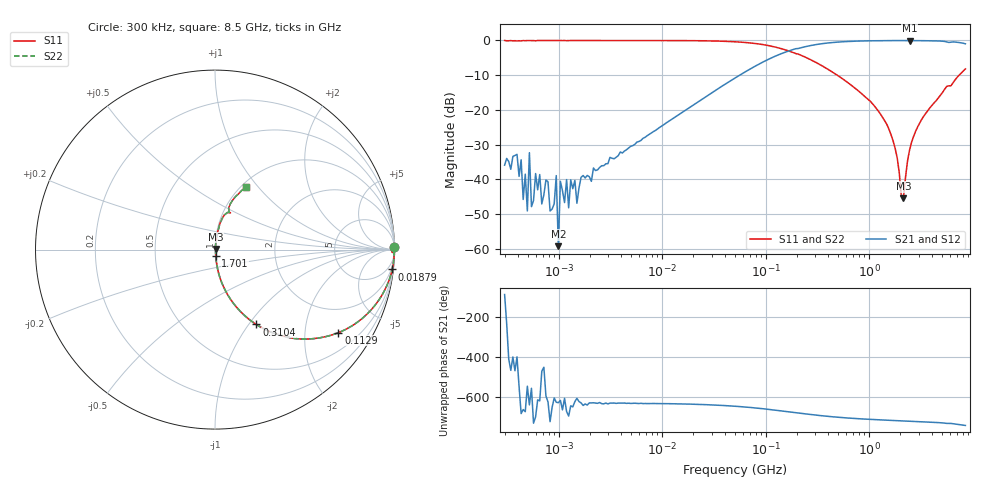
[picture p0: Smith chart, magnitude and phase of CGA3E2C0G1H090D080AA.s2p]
! S-parameter Generated by TDK Corporation
! Copyright(C) 2015 TDK Corporation.
! All Rights Reserved.
! TDK P/N: CGA3E2C0G1H090D080AA (Multilayer Ceramic Chip Capacitors)
! Property: C=9pF
! Size(LxWxT): 1.6x0.8x0.8mm, 0.063x0.031x0.031inches
! Model Type: s2p (Touchstone File Format Version 1.0)
! Frequency: DC=Yes Start=0.3MHz Stop=8500MHz 225points Log-sweep
! Note:
! Model Generated on Jun. 23, 2015
! Hash(MD5):
! Port Assignments:
!  1 ---| |--- 2
! Applicable Conditions:
!  Temperature = 25 degC
!  DC Bias Voltage = 0 V
!  Small Signal Operation
! Terms and conditions regarding TDK Simulation Models
! (1)This simulation model is being provided solely for informational purposes. Please refer to the specifications of the products in terms of detailed characteristics of such products.
! (2)In no event shall TDK Corporation of any of its subsidiaries be liable for any loss or damage arising, directly or indirectly,
!  From any information contained in this simulation model, including, but not limited to loss or damages arising from any inaccuracies, omissions or errors in connection with such information.
! (3)Any and all copyrights on this simulation model are owned by TDK Corporation.
!  Duplication or redistribution of this simulation model without prior written permission from TDK Corporation is prohibited.
! (4)This simulation model is subject to any modification or change without any prior notice.
! (5)Neither TDK Corporation nor any of its subsidiaries shall make any warranty, express or implied,
!  Including but not limited to the correctness, implied warranties of merchantability and fitness for a particular purpose with respect to this simulation models.
! (6)The use of this simulation model shall be deemed to have consented to the terms and conditions hereof.
# MHz S MA R 50
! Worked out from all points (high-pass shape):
!   224 points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, 300 kHz to 8.5 GHz, reference 50 ohm
!   highest |S21| = -0.03 dB at 2.457 GHz (marker M1); lowest = -59.3 dB at 991.3 kHz (marker M2)
!   |S21| within 3 dB of the highest: 166.8 MHz to end of sweep
!   lowest |S11| = -45.5 dB at 2.14 GHz (marker M3), VSWR 1.01, Z = 50.4 + j0.33 ohm
!   |S11| at or under -10 dB: 490.5 MHz to 7.398 GHz (6.908 GHz wide, 175 % of centre)
!   |S22| runs from -45.5 to 0.0 dB; largest |S21 - S12| = 9.6e-12
!   S11 on the Smith chart (normalised r, x): 300 kHz: open; 18.79 MHz: 1, -18; 112.9 MHz: 1.00, -2.97; 310.4 MHz: 1.01, -1.09; 1.701 GHz: 1.01, -0.07; 8.5 GHz: 1.06, +0.87
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0.3  0.9999 0.9  0.01597 -89.1  0.01597 -89.1  0.9999 0.9
0.4333561  0.9847 -0.7  0.0191 36.5  0.0191 36.5  0.9847 -0.7
0.4974407  0.9965 -0.0  0.0035 173.2  0.0035 173.2  0.9965 -0.0
0.5208429  0.996 -1.4  0.02418 79.9  0.02418 79.9  0.996 -1.4
0.5453461  0.9961 -0.0  0.004038 162.8  0.004038 162.8  0.9961 -0.0
0.8636283  0.9986 -0.2  0.003734 67.7  0.003734 67.7  0.9986 -0.2
0.9467989  0.9992 -0.6  0.0113 93.1  0.0113 93.1  0.9992 -0.6
0.9913414  1 -0.0  0.001088 90.8  0.001088 90.8  1 -0.0
1.037979  0.9979 -0.5  0.009351 102.1  0.009351 102.1  0.9979 -0.5
1.247529  0.9965 -0.1  0.003883 24.2  0.003883 24.2  0.9965 -0.1
1.72111  0.9975 -0.6  0.01133 77.1  0.01133 77.1  0.9975 -0.6
9.430415  0.998 -3.2  0.05586 86.4  0.05586 86.4  0.998 -3.2
18.79372  0.9937 -6.4  0.1111 83.6  0.1111 83.6  0.9937 -6.4
51.67171  0.9553 -17.1  0.2938 72.8  0.2938 72.8  0.9553 -17.1
112.8926  0.8285 -34.0  0.5587 55.9  0.5587 55.9  0.8285 -34.0
283.1228  0.5123 -58.7  0.8546 30.8  0.8546 30.8  0.5123 -58.7
310.3886  0.4767 -61.1  0.8751 28.5  0.8751 28.5  0.4767 -61.1
1551.304  0.05271 -83.8  0.9957 3.0  0.9957 3.0  0.05271 -83.8
1700.7  0.03589 -83.3  0.9964 2.1  0.9964 2.1  0.03589 -83.3
2140.204  0.005336 37.9  0.9958 -0.2  0.9958 -0.2  0.005336 37.9
2456.696  0.02658 82.5  0.9969 -1.5  0.9969 -1.5  0.02658 82.5
8500  0.3892 63.2  0.8948 -22.8  0.8948 -22.8  0.3892 63.2
